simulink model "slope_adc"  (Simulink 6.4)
settings: Solver=ode45  StartTime=0.0  StopTime=(kmod+nmod)/fmod  RelTol=1e-3
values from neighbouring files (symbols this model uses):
  acmag = 0.5    [go_slope_adc.m]
  F1 = 40E3    (= 40000)    [go_slope_adc.m]
  fmod = 8E3    (= 8000)    [go_slope_adc.m]
  tQ = 1/(2*osr*fmod)    (= 9.765625e-07)    [go_slope_adc.m]
undefined symbols (not defined in the file or in its folder): fq
libraries: simulink x1

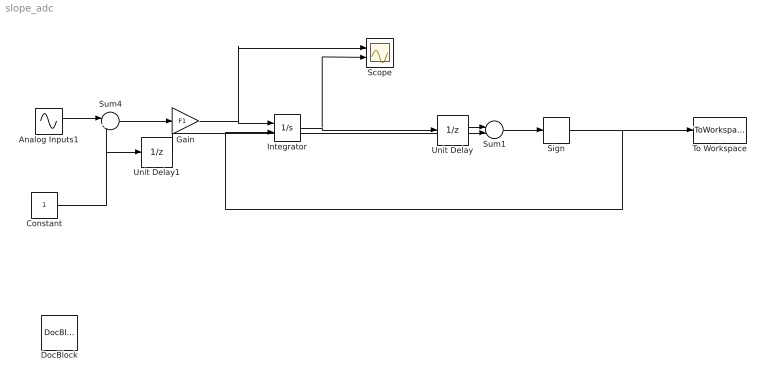
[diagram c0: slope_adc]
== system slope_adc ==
  Analog Inputs1 : Sin  Amplitude=acmag  Frequency=2*pi*fmod  Samples=round(fq/fmod)  SampleTime=tQ
  Constant : Constant
  DocBlock : simulink/Model-Wide Utilities/DocBlock  SystemSampleTime=-1  DocumentType=Text
  Gain : Gain  Gain=F1
  Integrator : Integrator  ExternalReset=falling
  Scope : Scope  NumInputPorts=2
  Sign : Signum
  Sum1 : Sum  Inputs=|-+
  Sum4 : Sum  Inputs=|++
  To Workspace : ToWorkspace  VariableName=yout  SampleTime=tQ  SaveFormat=Array
  Unit Delay : UnitDelay  SampleTime=tQ
  Unit Delay1 : UnitDelay  SampleTime=tQ
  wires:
  Analog Inputs1/1 -> Sum4/1
  Sign/1 -> To Workspace/1, Integrator/2
  Integrator/1 -> Scope/2, Unit Delay/1
  Sum4/1 -> Gain/1
  Constant/1 -> Sum4/2, Unit Delay1/1
  Unit Delay/1 -> Sum1/1
  Sum1/1 -> Sign/1
  Unit Delay1/1 -> Sum1/2
  Gain/1 -> Integrator/1, Scope/1
